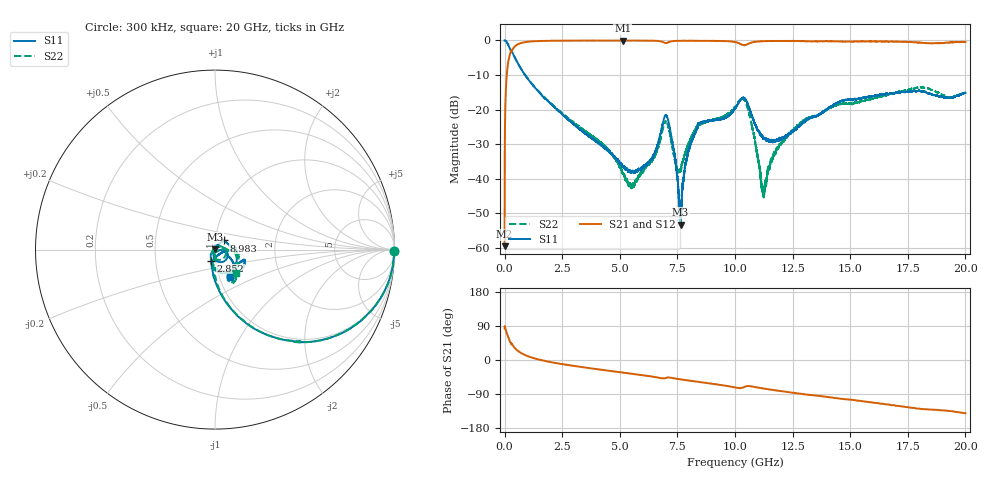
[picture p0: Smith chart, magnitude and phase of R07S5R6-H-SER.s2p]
!{R07S5R6}
!Johanson Technology Inc.
!www.johansontechnology.com
!Test Board Conditions:
!Substrate Type  RO4350B
!Substrate Thickness  10 mil
!Substrate Dk  3.66
!TL Type: GCPW
!TL Trace Width  21 mil
!TL Gap  20 mil
!Electrode orientation  Horizontal
!DUT TOPOLOGY	SERIES
!Mounting Pad LxW  16x21 mil
! Created Sat Feb  6 11:36:15 2021
# hz S ma R 50
! 2 Port Network Data from SP1.SP block
! freq  magS11  angS11  magS21  angS21  magS12  angS12  magS22  angS22
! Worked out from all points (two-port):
!   20001 points, 300 kHz to 20 GHz, reference 50 ohm
!   highest |S21| = -0.03 dB at 5.124 GHz (marker M1); lowest = -59.5 dB at 300 kHz (marker M2)
!   |S21| within 3 dB of the highest: 280.5 MHz to 299.9 MHz (19.4 MHz wide, 6.68 % of centre); 310 MHz to end of sweep
!   lowest |S11| = -53.2 dB at 7.636 GHz (marker M3), VSWR 1.00, Z = 49.8 + j0.0975 ohm
!   |S11| at or under -10 dB: 887.8 MHz to end of sweep
!   |S22| runs from -45.4 to 0.0 dB; largest |S21 - S12| = 0.011
!   S11 on the Smith chart (normalised r, x): 300 kHz: open; 2.852 GHz: 0.95, -0.12; 8.983 GHz: 1.09, +0.11; 20 GHz: 1.12, -0.36
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300000  1 -0.4  0.001063 83.4  0.001133 87.5  0.9998 -0.6
1.113e8  0.9267 -22.5  0.3697 67.8  0.3705 67.7  0.9279 -22.4
2.983e8  0.6793 -49.3  0.7258 41.4  0.7265 41.3  0.6808 -49.1
9.633e8  0.292 -78.9  0.9532 11.1  0.9538 11.0  0.2943 -78.2
2.8523e9  0.06767 -109.4  0.9945 -14.2  0.994 -14.2  0.07079 -95.0
3.3343e9  0.0498 -118.4  0.9953 -18.5  0.9956 -18.5  0.05382 -93.0
5.1243e9  0.01518 -118.8  0.9964 -33.1  0.995 -33.1  0.01174 -113.7
5.5593e9  0.01289 -83.3  0.9946 -36.6  0.9945 -36.6  0.008408 178.5
6.6673e9  0.03318 -2.1  0.9837 -46.4  0.9828 -46.4  0.02857 47.6
7.0723e9  0.07551 -67.9  0.9287 -46.1  0.9302 -46.2  0.06175 -68.4
7.4553e9  0.01392 -120.2  0.9861 -49.3  0.9865 -49.4  0.01491 -88.1
7.6363e9  0.002184 153.4  0.9882 -51.1  0.9892 -51.1  0.01344 -40.6
7.8833e9  0.01825 70.0  0.9896 -53.3  0.9896 -53.3  0.02605 -10.9
8.1523e9  0.03634 56.0  0.9892 -55.5  0.9893 -55.5  0.04372 -0.8
8.9833e9  0.07026 46.8  0.9855 -62.3  0.9861 -62.4  0.07022 -2.6
1.00003e10  0.103 -0.5  0.951 -72.4  0.9498 -72.4  0.1093 -7.7
1.05083e10  0.1307 -79.1  0.8729 -69.2  0.8732 -69.2  0.1153 -79.4
1.12363e10  0.03808 -81.1  0.974 -75.4  0.9776 -75.3  0.006679 139.3
1.18743e10  0.03546 -36.8  0.9822 -81.1  0.983 -81.0  0.0288 31.8
1.33343e10  0.07737 -23.4  0.9699 -92.7  0.9701 -92.7  0.07921 -6.5
1.66673e10  0.1668 -20.0  0.9571 -117.5  0.9608 -117.8  0.1662 -41.9
2e10  0.1747 -62.0  0.9549 -140.6  0.9496 -140.4  0.1772 -49.0
